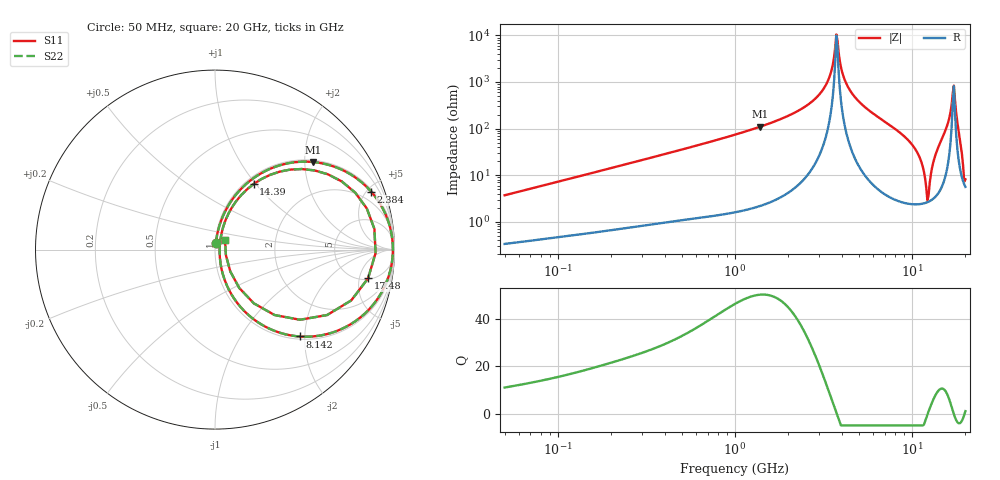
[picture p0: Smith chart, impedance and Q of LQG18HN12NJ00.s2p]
!Murata Part Number: LQG18HN12NJ00
!These Parameters are Measured in Series Mode Connection
!  o--[Z]--o
!Port1  Port2
!  o-------o
!Freq. Start=50[MHz] Stop=20[GHz], 401[Steps]
# Hz S RI R 50
!Freq.(Hz) S11(Real) S11(Imag) S21(Real) S21(Imag) S12(Real) S12(Imag) S22(Real) S22(Imag)
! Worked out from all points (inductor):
!   401 points, 50 MHz to 20 GHz, reference 50 ohm
!   read as one part in series: L = 11.6 nH near 51.52 MHz
!   highest Q = 50.3 at 1.39 GHz (marker M1), where L = 12.6 nH
!   self-resonance near 3.736 GHz
!   S11 on the Smith chart (normalised r, x): 50 MHz: 1.01, +0.07; 2.384 GHz: 1.15, +5.35; 8.142 GHz: 1.06, -1.88; 14.39 GHz: 1.09, +0.98; 17.48 GHz: 5.23, -6.78; 20 GHz: 1.11, +0.12
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5e7  0.00468 0.0365  0.9953 -0.0365  0.9953 -0.0365  0.00468 0.0365
1.364002e8  0.0147 0.0957  0.9853 -0.0957  0.9853 -0.0957  0.0147 0.0957
3.721004e8  0.0721 0.2416  0.9279 -0.2416  0.9279 -0.2416  0.0721 0.2416
1e9  0.3569 0.4684  0.6431 -0.4684  0.6431 -0.4684  0.3569 0.4684
1.390315e9  0.547 0.4879  0.453 -0.4879  0.453 -0.4879  0.547 0.4879
2.383959e9  0.8706 0.3222  0.1294 -0.3222  0.1294 -0.3222  0.8706 0.3222
2.728004e9  0.9287 0.2399  0.0713 -0.2399  0.0713 -0.2399  0.9287 0.2399
3.314454e9  0.9811 0.099  0.0189 -0.099  0.0189 -0.099  0.9811 0.099
3.736399e9  0.9911 0.00312  0.00893 -0.00312  0.00893 -0.00312  0.9911 0.00312
4.149438e9  0.9836 -0.0841  0.0164 0.0841  0.0164 0.0841  0.9836 -0.0841
4.608136e9  0.9593 -0.172  0.0407 0.172  0.0407 0.172  0.9593 -0.172
7.442007e9  0.5895 -0.478  0.4105 0.478  0.4105 0.478  0.5895 -0.478
8.141811e9  0.4709 -0.4841  0.5291 0.4841  0.5291 0.4841  0.4709 -0.4841
1.066139e10  0.1067 -0.2732  0.8933 0.2732  0.8933 0.2732  0.1067 -0.2732
1.220001e10  0.0257 -0.0117  0.9743 0.0117  0.9743 0.0117  0.0257 -0.0117
1.334722e10  0.0749 0.2003  0.9251 -0.2003  0.9251 -0.2003  0.0749 0.2003
1.438523e10  0.2154 0.3656  0.7846 -0.3656  0.7846 -0.3656  0.2154 0.3656
1.597544e10  0.6298 0.4193  0.3702 -0.4193  0.3702 -0.4193  0.6298 0.4193
1.696185e10  0.8882 0.1151  0.1118 -0.1151  0.1118 -0.1151  0.8882 0.1151
1.747767e10  0.8529 -0.16  0.1471 0.16  0.1471 0.16  0.8529 -0.16
1.855685e10  0.332 -0.3646  0.668 0.3646  0.668 0.3646  0.332 -0.3646
2e10  0.056 0.0527  0.944 -0.0527  0.944 -0.0527  0.056 0.0527
